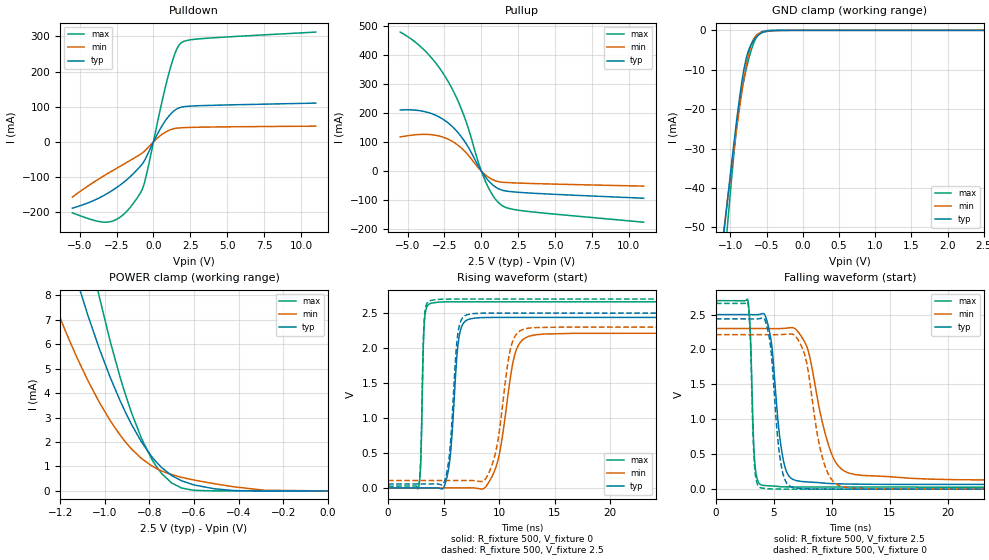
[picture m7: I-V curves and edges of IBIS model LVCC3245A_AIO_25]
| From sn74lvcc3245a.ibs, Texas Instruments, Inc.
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[Model]   LVCC3245A_AIO_25
Model_type  I/O
Vinl=0.7
Vinh=1.7
Enable   Active-Low
Vref =   0
Rref =   500
Cref =   30p
Vmeas =   1.25
| variable   typ   min   max
C_comp   18.50pF   NA   NA
| C_pullup   12.25pF   9.29pF   14.46pF
| C_pulldown   9.09pF   4.14pF   13.71pF
| C_tri-state   8.24pF   7.17pF   8.92pF
[Temperature Range]   40   100   -40
| Ambient temperature   25   85   -40
[Voltage range]   2.5   2.3   2.7
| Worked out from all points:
|   slope of the pulldown table from 0 to 0.375 V, typ, clamps not added: 12.2 ohm
|   slope of the pullup table from 0 to 0.375 V, typ, clamps not added: 14.1 ohm
|   GND clamp passes 1 mA (typ) near -0.60 V on its own axis
|   POWER clamp passes 1 mA (typ) near -0.75 V on its own axis
|   rising waveform, R_fixture 500, V_fixture 0: 20-80 % time 619ps typ, 1.26ns min, 222ps max; typ from 0 V to 2.44 V
|   falling waveform, R_fixture 500, V_fixture 2.5: 20-80 % time 832ps typ, 1.73ns min, 298ps max; typ from 2.5 V to 0.059 V
|   rising waveform, R_fixture 500, V_fixture 2.5: 20-80 % time 588ps typ, 1.13ns min, 218ps max; typ from 0.056 V to 2.5 V
|   falling waveform, R_fixture 500, V_fixture 0: 20-80 % time 723ps typ, 1.33ns min, 285ps max; typ from 2.44 V to 0 V
[GND Clamp]
| LVCC3245A_AIO_25
|   Voltage   I(typ)   I(min)   I(max)
-5.5V     -942.2mA   -838.7mA   -1.112A
-1.12V    -56.57mA   -54.91mA   -66.7mA
-1.075V   -48.86mA   -48.11mA   -56.82mA
-1.04V    -42.95mA   -42.9mA    -49.27mA
-930mV    -25.22mA   -27.07mA   -27.26mA
-890mV    -19.32mA   -21.65mA   -20.81mA
-850mV    -13.98mA   -16.54mA   -15.92mA
-780mV    -6.962mA   -8.755mA   -9.697mA
-715mV    -3.611mA   -3.734mA   -5.161mA
-645mV    -1.748mA   -1.296mA   -1.883mA
-580mV    -777.6uA   -575.6uA   -496.1uA
2.5V      1.311nA    3.05uA     21.69pA
[POWER Clamp]
| LVCC3245A_AIO_25
|   Voltage   I(typ)   I(min)   I(max)
-5.5V     377.9mA    260.8mA    635.5mA
-1.25V    12.75mA    8.244mA    18.97mA
-1.215V   11.52mA    7.41mA     16.99mA
-1.125V   8.607mA    5.457mA    12.34mA
-1.075V   7.156mA    4.496mA    10.04mA
-1.025V   5.828mA    3.629mA    7.952mA
-930mV    3.658mA    2.266mA    4.607mA
-835mV    1.996mA    1.323mA    2.138mA
-770mV    1.188mA    924uA      1.012mA
-700mV    627.1uA    664.4uA    322.5uA
-510mV    89.41uA    296.3uA    1.164uA
-95.1fV   1.311nA    9.355nA    24.38pA
[Pulldown]
| LVCC3245A_AIO_25
|   Voltage   I(typ)   I(min)   I(max)
-5.5V     -188.6mA   -157mA     -201.8mA
-3.8V     -161.9mA   -107.9mA   -225.7mA
-2.87V    -140.2mA   -84.25mA   -226.4mA
-1.95V    -112.6mA   -61.94mA   -203.4mA
-1.005V   -74.67mA   -38.37mA   -153.2mA
-565mV    -49.62mA   -24.63mA   -108.8mA
545mV     43.15mA    20.2mA     108.5mA
1.125V    77.37mA    34.16mA    207.2mA
1.54V     92.67mA    38.81mA    260.1mA
1.89V     98.77mA    40.19mA    282mA
3.29V     103.2mA    41.94mA    293.9mA
11V       110.4mA    44.78mA    312.4mA
[Pullup]
| LVCC3245A_AIO_25
|   Voltage   I(typ)   I(min)   I(max)
-5.5V     210.3mA    117.6mA    478.3mA
-3.745V   203.5mA    126.4mA    409.9mA
-2.97V    189mA      122mA      363.7mA
-2.275V   166.6mA    110.4mA    310.2mA
-1.705V   139.5mA    93.58mA    254.6mA
-1.195V   106.7mA    71.68mA    192.5mA
-185mV    15.79mA    10.35mA    27.19mA
245mV     -18.18mA   -11.64mA   -31.39mA
770mV     -47.43mA   -29.29mA   -83.22mA
1.305V    -63.84mA   -37.41mA   -114.8mA
2.895V    -74.13mA   -41.69mA   -137mA
11V       -93.18mA   -51.5mA    -175.6mA
[Ramp]
| LVCC3245A_AIO_25
| variable   typ   min   max
dV/dt_r   1.47/6.30E-10   1.34/1.27E-09   1.61/2.30E-10
dV/dt_f   1.47/8.36E-10   1.31/1.73E-09   1.62/3.07E-10
R_load = 500
[Rising Waveform]
| LVCC3245A_AIO_25
R_fixture =   500
C_fixture =   0
L_fixture =   0
V_fixture =   0
V_fixture_min = 0
V_fixture_max = 0
|   Time   V(typ)   V(min)   V(max)
0s        156pV      143.2nV    48.55pV
2.76ns    4.474uV    461nV      9.425mV
3.27ns    -9.039uV   -217.5nV   2.364V
3.86ns    -23.99uV   5.825uV    2.639V
5.33ns    169.8mV    -14.94uV   2.66V
6.345ns   2.101V     -28.55uV   2.661V
7.285ns   2.412V     1.542mV    2.661V
9.6ns     2.437V     243.2mV    2.661V
12.72ns   2.438V     2.17V      2.661V
50ns      2.438V     2.212V     2.661V
[Falling Waveform]
| LVCC3245A_AIO_25
R_fixture =   500
C_fixture =   0
L_fixture =   0
V_fixture =   2.5
V_fixture_min = 2.3
V_fixture_max = 2.7
|   Time   V(typ)   V(min)   V(max)
0s        2.5V       2.3V       2.7V
2.755ns   2.5V       2.3V       2.702V
3.335ns   2.498V     2.3V       416.2mV
3.9ns     2.508V     2.3V       61.05mV
4.74ns    2.15V      2.299V     45.56mV
5.825ns   410.9mV    2.302V     33.45mV
6.815ns   129mV      2.3V       31.42mV
9.95ns    80.36mV    521.7mV    30.67mV
11.56ns   73.23mV    225.7mV    30.64mV
50ns      59.44mV    126.4mV    25.56mV
[Rising Waveform]
| LVCC3245A_AIO_25
R_fixture =   500
C_fixture =   0
L_fixture =   0
V_fixture =   2.5
V_fixture_min = 2.3
V_fixture_max = 2.7
|   Time   V(typ)   V(min)   V(max)
0s        56.31mV    105.3mV    25.54mV
2.76ns    56.31mV    105.3mV    35.17mV
3.26ns    56.3mV     105.3mV    2.405V
3.82ns    56.29mV    105.3mV    2.68V
5.27ns    203.4mV    105.3mV    2.699V
6.275ns   2.186V     105.3mV    2.7V
7.135ns   2.477V     106.3mV    2.7V
9.31ns    2.499V     302.2mV    2.7V
12.23ns   2.5V       2.269V     2.7V
50ns      2.5V       2.3V       2.7V
[Falling Waveform]
| LVCC3245A_AIO_25
R_fixture =   500
C_fixture =   0
L_fixture =   0
V_fixture =   0
V_fixture_min = 0
V_fixture_max = 0
|   Time   V(typ)   V(min)   V(max)
0s        2.438V     2.212V     2.661V
2.75ns    2.438V     2.212V     2.664V
3.315ns   2.437V     2.212V     365.5mV
3.825ns   2.444V     2.212V     21.42mV
4.665ns   2.102V     2.211V     4.415mV
5.665ns   312.8mV    2.214V     949.2uV
6.58ns    28.8mV     2.221V     459.4uV
9.34ns    1.832mV    370.6mV    70.39uV
10.82ns   1.104mV    40.19mV    35.12uV
50ns      60.63uV    101.4uV    4.725uV
